PROGRAM MAIN_CM

VAR CONSTANT
	(* Histogram settings *)
	cInitHistArray		: ST_CM_HistArray_InitPars :=  (nChannels 	:= cChannels, 
														nBins 		:= cMaxBins, 
														fMinBinned 	:= cLowerBinLimit, 
														fMaxBinned 	:= cUpperBinLimit);
	(* settings for mean, std, skew, kurtosis *)														
	cInitMoments        : ST_CM_EmpiricalMoments_InitPars := (nChannels := cChannels);												
END_VAR

VAR
	(* Error monitoring *) 
	fbErrHist			: FB_HRErrHist;
	
	aMean				: ARRAY [1..cChannels] OF LREAL;	
	aStd           		: ARRAY [1..cChannels] OF LREAL;
	aSkewness      		: ARRAY [1..cChannels] OF LREAL;
	aExcessKurtosis		: ARRAY [1..cChannels] OF LREAL;

	(* Histogram *) 
	fbHistSink			: FB_CMA_Sink := (nOwnID := eID_Sink_Hist);			
	fbHistArray 		: FB_CMA_HistArray :=(stInitPars := cInitHistArray, nOwnID := eID_Histogram, aDestIDs := [eID_Sink_Hist]);
	
	// for each channel
	// -12 ... 12 spaced in 24/(cMaxBins-1); 
	// cMaxBins+1 = Number of values below LowerBinLimit;
	// cMaxBins+2 = Number of values over UpperBinLimit 
	aHistogram			: ARRAY [1..cChannels] OF ARRAY [1..cMaxBins+2] OF ULINT;
	aHistogram_NormDisp : ARRAY [1..cMaxBins+2] OF ULINT;
	aHistogram_GammaDisp: ARRAY [1..cMaxBins+2] OF ULINT;
	aHistogram_Sine     : ARRAY [1..cMaxBins+2] OF ULINT;

 	(* mean *)
	fbMeanSink			: FB_CMA_Sink := (nOwnID := eID_Sink_Mean);
	fbMean				: FB_CMA_EmpiricalMean :=(stInitPars := cInitMoments, nOwnID := eID_Mean, aDestIDs := [eID_Sink_Mean]);
	(* Standard Deviation *)
	fbStdSink			: FB_CMA_Sink := (nOwnID := eID_Sink_Std);
	fbStd				: FB_CMA_EmpiricalStandardDeviation :=(stInitPars := cInitMoments, nOwnID := eID_Std, aDestIDs := [eID_Sink_Std]);
	(* skewness *)
	fbSkewSink			: FB_CMA_Sink := (nOwnID := eID_Sink_Skew);
	fbSkew				: FB_CMA_EmpiricalSkew :=(stInitPars := cInitMoments, nOwnID := eID_Skew, aDestIDs := [eID_Sink_Skew]);	
	(* excess kurtosis *)
	fbExcessKurtSink	: FB_CMA_Sink := (nOwnID := eID_Sink_ExcessKurtosis);
	fbExcessKurtosis	: FB_CMA_EmpiricalExcess :=(stInitPars := cInitMoments, nOwnID := eID_ExcessKurtosis, aDestIDs := [eID_Sink_ExcessKurtosis]);
END_VAR


CallHistogram();	// Call Histogram and Sink

CallMean();			// Call Mean and Sink
CallStd();			// Call Std and Sink
CallSkew();			// Call Skew and Sink
CallExcess();		// Call Excess and Sink

aHistogram_NormDisp := aHistogram[1];
aHistogram_GammaDisp := aHistogram[2];
aHistogram_Sine := aHistogram[3];

ACTION CallExcess:

(* Excess Call *)
fbExcessKurtosis.CallEx(nAppendData := cAppendData, bResetData := TRUE);
IF fbExcessKurtosis.bError THEN
	fbErrHist.AddError(bErr := TRUE, hrErrCode := fbExcessKurtosis.hrErrorCode, sErrSource := 'MAIN_CM.fbExcessKurtosis');
	// ToDo: if error
END_IF

fbExcessKurtSink.Output1D(pDataOut 		:= ADR(aExcessKurtosis), 
						nDataOutSize 	:= SIZEOF(aExcessKurtosis), 
						eElementType 	:= eMA_TypeCode_LREAL, 
						nWorkDim 		:= 0,
						nElements 		:= 0,
						pStartIndex 	:= 0,					
						nOptionPars		:= 0);
IF fbExcessKurtSink.bError THEN
	fbErrHist.AddError(bErr := TRUE, hrErrCode := fbExcessKurtSink.hrErrorCode, sErrSource := 'MAIN_CM.fbExcessKurtSink'); 
	// ToDo: if error
END_IF
END_ACTION

ACTION CallHistogram:

(* Histogram Call *)
fbHistArray.CallEx(nAppendData := cAppendData, bResetData := TRUE);
IF fbHistArray.bError THEN
	fbErrHist.AddError(bErr := TRUE, hrErrCode := fbHistArray.hrErrorCode, sErrSource := 'MAIN_CM.fbHistArray');
	// ToDo: if error
END_IF

fbHistSink.Output2D(pDataOut 		:= ADR(aHistogram), 
					nDataOutSize 	:= SIZEOF(aHistogram), 
					eElementType 	:= eMA_TypeCode_UINT64, 
					nWorkDim0 		:= 0,
					nWorkDim1 		:= 1,
					nElementsDim0 	:= 0,
					nElementsDim1 	:= 0,
					pStartIndex 	:= 0,					
					nOptionPars		:= 0,
					bNewResult  =>    );			
IF fbHistSink.bError THEN
	fbErrHist.AddError(bErr := TRUE, hrErrCode := fbHistSink.hrErrorCode, sErrSource := 'MAIN_CM.fbHistSink'); 
	// ToDo: if error
END_IF
END_ACTION

ACTION CallMean:

(* Mean Call *)
fbMean.CallEx(nAppendData := cAppendData, bResetData := TRUE);
IF fbMean.bError THEN
	fbErrHist.AddError(bErr := TRUE, hrErrCode := fbMean.hrErrorCode, sErrSource := 'MAIN_CM.fbMean');
	// ToDo: if error
END_IF

fbMeanSink.Output1D(pDataOut 		:= ADR(aMean), 
					nDataOutSize 	:= SIZEOF(aMean), 
					eElementType 	:= eMA_TypeCode_LREAL, 
					nWorkDim 		:= 0,
					nElements 		:= 0,
					pStartIndex 	:= 0,					
					nOptionPars		:= 0);			
IF fbMeanSink.bError THEN
	fbErrHist.AddError(bErr := TRUE, hrErrCode := fbMeanSink.hrErrorCode, sErrSource := 'MAIN_CM.fbMeanSink'); 
	// ToDo: if error
END_IF
END_ACTION

ACTION CallSkew:

(* Skew Call *)
fbSkew.CallEx(nAppendData := cAppendData, bResetData := TRUE);
IF fbSkew.bError THEN
	fbErrHist.AddError(bErr := TRUE, hrErrCode := fbSkew.hrErrorCode, sErrSource := 'MAIN_CM.fbSkew');
	// ToDo: if error
END_IF

fbSkewSink.Output1D(pDataOut 		:= ADR(aSkewness), 
					nDataOutSize 	:= SIZEOF(aSkewness), 
					eElementType 	:= eMA_TypeCode_LREAL, 
					nWorkDim 		:= 0,
					nElements 		:= 0,
					pStartIndex 	:= 0,					
					nOptionPars		:= 0);
IF fbSkewSink.bError THEN
	fbErrHist.AddError(bErr := TRUE, hrErrCode := fbSkewSink.hrErrorCode, sErrSource := 'MAIN_CM.fbSkewSink'); 
	// ToDo: if error
END_IF
END_ACTION

ACTION CallStd:

(* Std Call *)
fbStd.CallEx(nAppendData := cAppendData, bResetData := TRUE);
IF fbStd.bError THEN
	fbErrHist.AddError(bErr := TRUE, hrErrCode := fbStd.hrErrorCode, sErrSource := 'MAIN_CM.fbStd');
	// ToDo: if error
END_IF

fbStdSink.Output1D(pDataOut 		:= ADR(aStd), 
					nDataOutSize 	:= SIZEOF(aStd), 
					eElementType 	:= eMA_TypeCode_LREAL, 
					nWorkDim 		:= 0,
					nElements 		:= 0,
					pStartIndex 	:= 0,					
					nOptionPars		:= 0);			
IF fbStdSink.bError THEN
	fbErrHist.AddError(bErr := TRUE, hrErrCode := fbStdSink.hrErrorCode, sErrSource := 'MAIN_CM.fbStdSink'); 
	// ToDo: if error
END_IF
END_ACTION

END_PROGRAM
